VAR_GLOBAL CONSTANT
	MIN_SLAVES												: 	UINT  := 1;
	MAX_SLAVES												: 	UINT  := 1000;
	MIN_ANALOGVALUE											:	LREAL := 0;
	MAX_ANALOGVALUE											:	LREAL := 32767;
	TimeZone                 							    :   INT   := 30;			// FB_SignalAlarmRecord
	MaxReadSizeBuff											: UDINT		:= 1024;
END_VAR
